| IBIS file stm32h562_563_573_lqfp100.ibs
[IBIS ver] 4.2
[File name] stm32h562_563_573_lqfp100.ibs
[File Rev] 1.1
[Date] 07-05-2024
[Source] Data Created at STMicroelectronics
[Notes]  File originated from ELDO simulations.
[Disclaimer]  This information is for modeling purpose only and is
   not guaranteed. The information is subject to change without
   notice.
[Copyright] Copyright 2024 STMicroelectronics Inc.
|   Component stm32h562_563_573_lqfp100
[Component] stm32h562_563_573_lqfp100
[Manufacturer] STMicroelectronics
[Package]
| variable   typ   min   max
R_pkg  0  NA  NA
L_pkg  0  NA  NA
C_pkg  0  NA  NA
[Pin]   signal_name   model_name
1  PE2  io8_ft_i3c_spi
2  PE3  io8_ft_i3c_spi
3  PE4  io8_ft_i3c_spi
4  PE5  io8_ft_i3c_spi
5  PE6  io8_ft_i3c_spi
6  VBAT  power
7  PC13  io8_ft_i3c_spi
8  PC14-OSC32_IN  io8_ft_i3c_spi
9  PC15-OSC32_OUT  io8_ft_i3c_spi
10  VSS  gnd
11  VDD  power
12  PH0-OSC_IN  io8_ft_i3c_spi
13  PH1-OSC_OUT  io8_ft_i3c_spi
14  NRST  ioreset_ft_v33
15  PC0  io8_ft_spi
16  PC1  io8_ft_spi
17  PC2  io8_ft_spi
18  PC3  io8_ft_spi
19  VSSA  nc
20  VREFM  nc
21  VREFP  nc
22  VDDA  nc
23  PA0  io8_ft_spi
24  PA1  io8_ft_spi_tamp
25  PA2  io8_ft_spi
26  PA3  io8_ft_spi
27  VSS  gnd
28  VDD  power
29  PA4  io8_ft_spi
30  PA5  io8_ft_spi
31  PA6  io8_ft_spi
32  PA7  io8_ft_spi
33  PC4  io8_ft_spi
34  PC5  io8_ft_spi
35  PB0  io8_ft_spi
36  PB1  io8_ft_spi
37  PB2  io8_ft_i3c_spi
38  PE7  io8_ft_i3c_spi
39  PE8  io8_ft_i3c_spi
40  PE9  io8_ft_i3c_spi
41  PE10  io8_ft_i3c_spi
42  PE11  io8_ft_i3c_spi
43  PE12  io8_ft_i3c_spi
44  PE13  io8_ft_i3c_spi
45  PE14  io8_ft_i3c_spi
46  PE15  io8_ft_i3c_spi
47  PB10  io8_ft_i3c_spi
48  VCAP  nc
49  VSS  gnd
50  VDD  power
51  PB12  io8_ft_i3c_spi
52  PB13  nc
|io8usb_ft_pd
53  PB14  nc
|io8usb_ft_pd
54  PB15  io8_ft_spi
55  PD8  io8_ft_i3c_spi
56  PD9  io8_ft_i3c_spi
57  PD10  io8_ft_i3c_spi
58  PD11  io8_ft_i3c_spi
59  PD12  io8_ft_i3c_spi
60  PD13  io8_ft_i3c_spi
61  PD14  io8_ft_i3c_spi
62  PD15  io8_ft_i3c_spi
63  PC6  io8_ft_i3c_spi
64  PC7  io8_ft_i3c_spi
65  PC8  io8_ft_i3c_spi
66  PC9  io8_ft_i3c_spi
67  PA8  io8_ft_i3c_spi
68  PA9  io8_ft_i3c_spi
69  PA10  io8_ft_i3c_spi
70  PA11  io8usb_ft_i3c_spi_phy
71  PA12  io8usb_ft_i3c_spi_phy
72  PA13  io8_ft_i3c_spi
73  VDD33_USB  power
74  VSS  gnd
75  VDD  power
76  PA14  io8_ft_i3c_spi
77  PA15  io8_ft_i3c_spi
78  PC10  io8_ft_i3c_spi
79  PC11  io8_ft_i3c_spi
80  PC12  io8_ft_i3c_spi
81  PD0  io8_ft_i3c_spi
82  PD1  io8_ft_i3c_spi
83  PD2  io8_ft_i3c_spi
84  PD3  io8_ft_i3c_spi
85  PD4  io8_ft_i3c_spi
86  PD5  io8_ft_i3c_spi
87  PD6  io8_ft_i3c_spi
88  PD7  io8_ft_i3c_spi
89  PB3  io8_ft_i3c_spi
90  PB4  io8_ft_i3c_spi
91  PB5  io8_ft_i3c_spi
92  PB6  io8_ft_i3c_spi
93  PB7  io8_ft_i3c_spi
94  BOOT0  vpphv
95  PB8  io8_ft_i3c_spi
96  PB9  io8_ft_i3c_spi
97  PE0  io8_ft_i3c_spi
98  VCAP  nc
99  VSS  gnd
100  VDD  power
[Package Model]   484-lqfp-14x14-100-ldo-221014
[Pin Mapping]   pulldown_ref   pullup_ref   | Comment
1  gndio  vddiom
2  gndio  vddiom
3  gndio  vddiom
4  gndio  vddiom
5  gndio  vddiom
6  nc  vsw
7  gndio  vddiom  | Depending on IO usage
| 7  gndio  vsw  | Depending on IO usage
8  gndio  vddiom  | Depending on IO usage
| 8  gndio  vsw  | Depending on IO usage
9  gndio  vddiom  | Depending on IO usage
| 9  gndio  vsw  | Depending on IO usage
10  gndio  nc
11  nc  vddiom
12  gndio  vddiom
13  gndio  vddiom
14  gndio  vddiom
15  gndio  vddiom
16  gndio  vddiom
17  gndio  vddiom
18  gndio  vddiom
19  nc  nc
20  nc  nc
21  nc  nc
22  nc  nc
23  gndio  vddiom
24  gndio  vddiom
25  gndio  vddiom
26  gndio  vddiom
27  gndio  nc
28  nc  vddiom
29  gndio  vddiom
30  gndio  vddiom
31  gndio  vddiom
32  gndio  vddiom
33  gndio  vddiom
34  gndio  vddiom
35  gndio  vddiom
36  gndio  vddiom
37  gndio  vddiom
38  gndio  vddiom
39  gndio  vddiom
40  gndio  vddiom
41  gndio  vddiom
42  gndio  vddiom
43  gndio  vddiom
44  gndio  vddiom
45  gndio  vddiom
46  gndio  vddiom
47  gndio  vddiom
48  nc  nc
49  gndio  nc
50  nc  vddiom
51  gndio  vddiom
|52  gndio  vddiom
|53  gndio  vddiom
52  nc  nc
53  nc  nc
54  gndio  vddiom
55  gndio  vddiom
56  gndio  vddiom
57  gndio  vddiom
58  gndio  vddiom
59  gndio  vddiom
60  gndio  vddiom
61  gndio  vddiom
62  gndio  vddiom
63  gndio  vddiom
64  gndio  vddiom
65  gndio  vddiom
66  gndio  vddiom
67  gndio  vddiom
68  gndio  vddiom  | Depending on IO usage
| 68  gndio  vddusb  | Depending on IO usage
69  gndio  vddiom  | Depending on IO usage
| 69  gndio  vddusb  | Depending on IO usage
70  gndio  vddiom  | Depending on IO usage
| 70  gndio  vddusb  | Depending on IO usage
71  gndio  vddiom  | Depending on IO usage
| 71  gndio  vddusb  | Depending on IO usage
72  gndio  vddiom  | Depending on IO usage
| 72  gndio  vddusb  | Depending on IO usage
73  nc  vddusb
74  gndio  nc
75  nc  vddiom
76  gndio  vddiom
77  gndio  vddiom
78  gndio  vddiom
79  gndio  vddiom
80  gndio  vddiom
81  gndio  vddiom
82  gndio  vddiom
83  gndio  vddiom
84  gndio  vddiom
85  gndio  vddiom
86  gndio  vddiom
87  gndio  vddiom
88  gndio  vddiom
89  gndio  vddiom
90  gndio  vddiom
91  gndio  vddiom
92  gndio  vddiom
93  gndio  vddiom
94  gndio  vddiom
95  gndio  vddiom
96  gndio  vddiom
97  gndio  vddiom
98  nc  nc
99  gndio  nc
100  nc  vddiom
[Model Selector] io8_ft_i3c_spi
io8_ft_spi_ls_1v2 "io8_ft spi low speed @ 1.2V"
io8_ft_spi_ls_1v8 "io8_ft spi low speed @ 1.8V"
io8_ft_spi_ls_3v3 "io8_ft spi low speed @ 3.3V"
io8_ft_spi_ms_1v2 "io8_ft spi med speed @ 1.2V"
io8_ft_spi_ms_1v8 "io8_ft spi med speed @ 1.8V"
io8_ft_spi_ms_3v3 "io8_ft spi med speed @ 3.3V"
io8_ft_spi_fs_1v2 "io8_ft spi fast speed @ 1.2V"
io8_ft_spi_fs_1v8 "io8_ft spi fast speed @ 1.8V"
io8_ft_spi_fs_3v3 "io8_ft spi fast speed @ 3.3V"
io8_ft_spi_hs_1v2 "io8_ft spi high speed @ 1.2V"
io8_ft_spi_hs_1v8 "io8_ft spi high speed @ 1.8V"
io8_ft_spi_hs_3v3 "io8_ft spi high speed @ 3.3V"
io8_ft_hslv_spi_ls_1v2 "io8_ft spi hslv low speed @ 1.2V"
io8_ft_hslv_spi_ls_1v8 "io8_ft spi hslv low speed @ 1.8V"
io8_ft_hslv_spi_ls_2v5 "io8_ft spi hslv low speed @ 2.5V"
io8_ft_hslv_spi_ms_1v2 "io8_ft spi hslv med speed @ 1.2V"
io8_ft_hslv_spi_ms_1v8 "io8_ft spi hslv med speed @ 1.8V"
io8_ft_hslv_spi_ms_2v5 "io8_ft spi hslv med speed @ 2.5V"
io8_ft_hslv_spi_fs_1v2 "io8_ft spi hslv fast speed @ 1.2V"
io8_ft_hslv_spi_fs_1v8 "io8_ft spi hslv fast speed @ 1.8V"
io8_ft_hslv_spi_fs_2v5 "io8_ft spi hslv fast speed @ 2.5V"
io8_ft_hslv_spi_hs_1v2 "io8_ft spi hslv high speed @ 1.2V"
io8_ft_hslv_spi_hs_1v8 "io8_ft spi hslv high speed @ 1.8V"
io8_ft_hslv_spi_hs_2v5 "io8_ft spi hslv high speed @ 2.5V"
io8_ft_i3c_spi_ls_1v2 "io8_ft i3c spi open-drain low speed @ 1.2V"
io8_ft_i3c_spi_ls_1v8 "io8_ft i3c spi open-drain low speed @ 1.8V"
io8_ft_i3c_spi_ls_3v3 "io8_ft i3c spi open-drain low speed @ 3.3V"
io8_ft_i3c_spi_ms_1v2 "io8_ft i3c spi open-drain med speed @ 1.2V"
io8_ft_i3c_spi_ms_1v8 "io8_ft i3c spi open-drain med speed @ 1.8V"
io8_ft_i3c_spi_ms_3v3 "io8_ft i3c spi open-drain med speed @ 3.3V"
io8_ft_i3c_spi_fs_1v2 "io8_ft i3c spi open-drain fast speed @ 1.2V"
io8_ft_i3c_spi_fs_1v8 "io8_ft i3c spi open-drain fast speed @ 1.8V"
io8_ft_i3c_spi_fs_3v3 "io8_ft i3c spi open-drain fast speed @ 3.3V"
io8_ft_i3c_spi_hs_1v2 "io8_ft i3c spi open-drain high speed @ 1.2V"
io8_ft_i3c_spi_hs_1v8 "io8_ft i3c spi open-drain high speed @ 1.8V"
io8_ft_i3c_spi_hs_3v3 "io8_ft i3c spi open-drain high speed @ 3.3V"
io8_ft_hslv_i3c_spi_ls_1v2 "io8_ft hslv i3c spi open-drain low speed @ 1.2V"
io8_ft_hslv_i3c_spi_ls_1v8 "io8_ft hslv i3c spi open-drain low speed @ 1.8V"
io8_ft_hslv_i3c_spi_ls_2v5 "io8_ft hslv i3c spi open-drain low speed @ 2.5V"
io8_ft_hslv_i3c_spi_ms_1v2 "io8_ft hslv i3c spi open-drain med speed @ 1.2V"
io8_ft_hslv_i3c_spi_ms_1v8 "io8_ft hslv i3c spi open-drain med speed @ 1.8V"
io8_ft_hslv_i3c_spi_ms_2v5 "io8_ft hslv i3c spi open-drain med speed @ 2.5V"
io8_ft_hslv_i3c_spi_fs_1v2 "io8_ft hslv i3c spi open-drain fast speed @ 1.2V"
io8_ft_hslv_i3c_spi_fs_1v8 "io8_ft hslv i3c spi open-drain fast speed @ 1.8V"
io8_ft_hslv_i3c_spi_fs_2v5 "io8_ft hslv i3c spi open-drain fast speed @ 2.5V"
io8_ft_hslv_i3c_spi_hs_1v2 "io8_ft hslv i3c spi open-drain high speed @ 1.2V"
io8_ft_hslv_i3c_spi_hs_1v8 "io8_ft hslv i3c spi open-drain high speed @ 1.8V"
io8_ft_hslv_i3c_spi_hs_2v5 "io8_ft hslv i3c spi open-drain high speed @ 2.5V"
io8_ft_i3c_fmp_spi_3v3 "io8_ft i3c fm+ spi open-drain @ 3.3V"
io8_ft_i3c_fmp_spi_1v8 "io8_ft i3c fm+ spi open-drain @ 1.8V"
io8_ft_i3c_fmp_spi_1v2 "io8_ft i3c fm+ spi open-drain @ 1.2V"
[Model Selector] io8_ft_spi
io8_ft_spi_ls_1v2 "io8_ft spi low speed @ 1.2V"
io8_ft_spi_ls_1v8 "io8_ft spi low speed @ 1.8V"
io8_ft_spi_ls_3v3 "io8_ft spi low speed @ 3.3V"
io8_ft_spi_ms_1v2 "io8_ft spi med speed @ 1.2V"
io8_ft_spi_ms_1v8 "io8_ft spi med speed @ 1.8V"
io8_ft_spi_ms_3v3 "io8_ft spi med speed @ 3.3V"
io8_ft_spi_fs_1v2 "io8_ft spi fast speed @ 1.2V"
io8_ft_spi_fs_1v8 "io8_ft spi fast speed @ 1.8V"
io8_ft_spi_fs_3v3 "io8_ft spi fast speed @ 3.3V"
io8_ft_spi_hs_1v2 "io8_ft spi high speed @ 1.2V"
io8_ft_spi_hs_1v8 "io8_ft spi high speed @ 1.8V"
io8_ft_spi_hs_3v3 "io8_ft spi high speed @ 3.3V"
io8_ft_hslv_spi_ls_1v2 "io8_ft spi hslv low speed @ 1.2V"
io8_ft_hslv_spi_ls_1v8 "io8_ft spi hslv low speed @ 1.8V"
io8_ft_hslv_spi_ls_2v5 "io8_ft spi hslv low speed @ 2.5V"
io8_ft_hslv_spi_ms_1v2 "io8_ft spi hslv med speed @ 1.2V"
io8_ft_hslv_spi_ms_1v8 "io8_ft spi hslv med speed @ 1.8V"
io8_ft_hslv_spi_ms_2v5 "io8_ft spi hslv med speed @ 2.5V"
io8_ft_hslv_spi_fs_1v2 "io8_ft spi hslv fast speed @ 1.2V"
io8_ft_hslv_spi_fs_1v8 "io8_ft spi hslv fast speed @ 1.8V"
io8_ft_hslv_spi_fs_2v5 "io8_ft spi hslv fast speed @ 2.5V"
io8_ft_hslv_spi_hs_1v2 "io8_ft spi hslv high speed @ 1.2V"
io8_ft_hslv_spi_hs_1v8 "io8_ft spi hslv high speed @ 1.8V"
io8_ft_hslv_spi_hs_2v5 "io8_ft spi hslv high speed @ 2.5V"
[Model Selector] io8_ft_spi_tamp
io8_ft_spi_ls_1v2 "io8_ft spi low speed @ 1.2V"
io8_ft_spi_ls_1v8 "io8_ft spi low speed @ 1.8V"
io8_ft_spi_ls_3v3 "io8_ft spi low speed @ 3.3V"
io8_ft_spi_ms_1v2 "io8_ft spi med speed @ 1.2V"
io8_ft_spi_ms_1v8 "io8_ft spi med speed @ 1.8V"
io8_ft_spi_ms_3v3 "io8_ft spi med speed @ 3.3V"
io8_ft_spi_fs_1v2 "io8_ft spi fast speed @ 1.2V"
io8_ft_spi_fs_1v8 "io8_ft spi fast speed @ 1.8V"
io8_ft_spi_fs_3v3 "io8_ft spi fast speed @ 3.3V"
io8_ft_spi_hs_1v2 "io8_ft spi high speed @ 1.2V"
io8_ft_spi_hs_1v8 "io8_ft spi high speed @ 1.8V"
io8_ft_spi_hs_3v3 "io8_ft spi high speed @ 3.3V"
io8_ft_hslv_spi_ls_1v2 "io8_ft spi hslv low speed @ 1.2V"
io8_ft_hslv_spi_ls_1v8 "io8_ft spi hslv low speed @ 1.8V"
io8_ft_hslv_spi_ls_2v5 "io8_ft spi hslv low speed @ 2.5V"
io8_ft_hslv_spi_ms_1v2 "io8_ft spi hslv med speed @ 1.2V"
io8_ft_hslv_spi_ms_1v8 "io8_ft spi hslv med speed @ 1.8V"
io8_ft_hslv_spi_ms_2v5 "io8_ft spi hslv med speed @ 2.5V"
io8_ft_hslv_spi_fs_1v2 "io8_ft spi hslv fast speed @ 1.2V"
io8_ft_hslv_spi_fs_1v8 "io8_ft spi hslv fast speed @ 1.8V"
io8_ft_hslv_spi_fs_2v5 "io8_ft spi hslv fast speed @ 2.5V"
io8_ft_hslv_spi_hs_1v2 "io8_ft spi hslv high speed @ 1.2V"
io8_ft_hslv_spi_hs_1v8 "io8_ft spi hslv high speed @ 1.8V"
io8_ft_hslv_spi_hs_2v5 "io8_ft spi hslv high speed @ 2.5V"
io8_ft_tamp_v33_1v2 "io8_ft tamp V33 @ 1.2V"
io8_ft_tamp_v33_1v8 "io8_ft tamp V33 @ 1.2V"
io8_ft_tamp_v33_3v3 "io8_ft tamp V33 @ 1.2V"
[Model Selector] io8usb_ft_i3c_spi_phy
io8_ft_spi_ls_1v2 "io8_ft spi low speed @ 1.2V"
io8_ft_spi_ls_1v8 "io8_ft spi low speed @ 1.8V"
io8_ft_spi_ls_3v3 "io8_ft spi low speed @ 3.3V"
io8_ft_spi_ms_1v2 "io8_ft spi med speed @ 1.2V"
io8_ft_spi_ms_1v8 "io8_ft spi med speed @ 1.8V"
io8_ft_spi_ms_3v3 "io8_ft spi med speed @ 3.3V"
io8_ft_spi_fs_1v2 "io8_ft spi fast speed @ 1.2V"
io8_ft_spi_fs_1v8 "io8_ft spi fast speed @ 1.8V"
io8_ft_spi_fs_3v3 "io8_ft spi fast speed @ 3.3V"
io8_ft_spi_hs_1v2 "io8_ft spi high speed @ 1.2V"
io8_ft_spi_hs_1v8 "io8_ft spi high speed @ 1.8V"
io8_ft_spi_hs_3v3 "io8_ft spi high speed @ 3.3V"
io8_ft_hslv_spi_ls_1v2 "io8_ft spi hslv low speed @ 1.2V"
io8_ft_hslv_spi_ls_1v8 "io8_ft spi hslv low speed @ 1.8V"
io8_ft_hslv_spi_ls_2v5 "io8_ft spi hslv low speed @ 2.5V"
io8_ft_hslv_spi_ms_1v2 "io8_ft spi hslv med speed @ 1.2V"
io8_ft_hslv_spi_ms_1v8 "io8_ft spi hslv med speed @ 1.8V"
io8_ft_hslv_spi_ms_2v5 "io8_ft spi hslv med speed @ 2.5V"
io8_ft_hslv_spi_fs_1v2 "io8_ft spi hslv fast speed @ 1.2V"
io8_ft_hslv_spi_fs_1v8 "io8_ft spi hslv fast speed @ 1.8V"
io8_ft_hslv_spi_fs_2v5 "io8_ft spi hslv fast speed @ 2.5V"
io8_ft_hslv_spi_hs_1v2 "io8_ft spi hslv high speed @ 1.2V"
io8_ft_hslv_spi_hs_1v8 "io8_ft spi hslv high speed @ 1.8V"
io8_ft_hslv_spi_hs_2v5 "io8_ft spi hslv high speed @ 2.5V"
io8_ft_i3c_spi_ls_1v2 "io8_ft i3c spi open-drain low speed @ 1.2V"
io8_ft_i3c_spi_ls_1v8 "io8_ft i3c spi open-drain low speed @ 1.8V"
io8_ft_i3c_spi_ls_3v3 "io8_ft i3c spi open-drain low speed @ 3.3V"
io8_ft_i3c_spi_ms_1v2 "io8_ft i3c spi open-drain med speed @ 1.2V"
io8_ft_i3c_spi_ms_1v8 "io8_ft i3c spi open-drain med speed @ 1.8V"
io8_ft_i3c_spi_ms_3v3 "io8_ft i3c spi open-drain med speed @ 3.3V"
io8_ft_i3c_spi_fs_1v2 "io8_ft i3c spi open-drain fast speed @ 1.2V"
io8_ft_i3c_spi_fs_1v8 "io8_ft i3c spi open-drain fast speed @ 1.8V"
io8_ft_i3c_spi_fs_3v3 "io8_ft i3c spi open-drain fast speed @ 3.3V"
io8_ft_i3c_spi_hs_1v2 "io8_ft i3c spi open-drain high speed @ 1.2V"
io8_ft_i3c_spi_hs_1v8 "io8_ft i3c spi open-drain high speed @ 1.8V"
io8_ft_i3c_spi_hs_3v3 "io8_ft i3c spi open-drain high speed @ 3.3V"
io8_ft_hslv_i3c_spi_ls_1v2 "io8_ft hslv i3c spi open-drain low speed @ 1.2V"
io8_ft_hslv_i3c_spi_ls_1v8 "io8_ft hslv i3c spi open-drain low speed @ 1.8V"
io8_ft_hslv_i3c_spi_ls_2v5 "io8_ft hslv i3c spi open-drain low speed @ 2.5V"
io8_ft_hslv_i3c_spi_ms_1v2 "io8_ft hslv i3c spi open-drain med speed @ 1.2V"
io8_ft_hslv_i3c_spi_ms_1v8 "io8_ft hslv i3c spi open-drain med speed @ 1.8V"
io8_ft_hslv_i3c_spi_ms_2v5 "io8_ft hslv i3c spi open-drain med speed @ 2.5V"
io8_ft_hslv_i3c_spi_fs_1v2 "io8_ft hslv i3c spi open-drain fast speed @ 1.2V"
io8_ft_hslv_i3c_spi_fs_1v8 "io8_ft hslv i3c spi open-drain fast speed @ 1.8V"
io8_ft_hslv_i3c_spi_fs_2v5 "io8_ft hslv i3c spi open-drain fast speed @ 2.5V"
io8_ft_hslv_i3c_spi_hs_1v2 "io8_ft hslv i3c spi open-drain high speed @ 1.2V"
io8_ft_hslv_i3c_spi_hs_1v8 "io8_ft hslv i3c spi open-drain high speed @ 1.8V"
io8_ft_hslv_i3c_spi_hs_2v5 "io8_ft hslv i3c spi open-drain high speed @ 2.5V"
io8_ft_i3c_fmp_spi_3v3 "io8_ft i3c fm+ spi open-drain @ 3.3V"
io8_ft_i3c_fmp_spi_1v8 "io8_ft i3c fm+ spi open-drain @ 1.8V"
io8_ft_i3c_fmp_spi_1v2 "io8_ft i3c fm+ spi open-drain @ 1.2V"
io8usb_ft_phy_ls_2v5 "iousb ft low speed @ 2.5V"
io8usb_ft_phy_ls_3v3 "iousb ft low speed @ 3.3V"
io8usb_ft_phy_fs_2v5 "iousb ft fast speed @ 2.5V"
io8usb_ft_phy_fs_3v3 "iousb ft fast speed @ 3.3V"
[Model Selector] ioreset_ft_v33
ioreset_ft_v33_1v2 "Reset PAD. 5V tolerant. 1.2V range"
ioreset_ft_v33_1v8 "Reset PAD. 5V tolerant. 1.8V range"
ioreset_ft_v33_3v3 "Reset PAD. 5V tolerant. 3.3V range"
[Model Selector] vpphv
vpphv_1v2 "Flash Test cell v33 = 1.2 V range"
vpphv_1v8 "Flash Test cell v33 = 1.8 V range"
vpphv_3v3 "Flash Test cell v33 = 3.3 V range"
[Define Package Model]  484-lqfp-14x14-100-ldo-221014
[Manufacturer]  Unknown
[OEM]  Unknown
[Description]  None
[Number Of Pins]  96
[Pin Numbers]
| Pin Num   Terminal Name
14 | NRST
23 | PA0
24 | PA1
25 | PA2
26 | PA3
29 | PA4
30 | PA5
31 | PA6
32 | PA7
67 | PA8
68 | PA9
69 | PA10
70 | PA11
71 | PA12
72 | PA13
76 | PA14
77 | PA15
35 | PB0
36 | PB1
37 | PB2
89 | PB3
90 | PB4
91 | PB5
92 | PB6
93 | PB7
95 | PB8
96 | PB9
47 | PB10
51 | PB12
52 | PB13
53 | PB14
54 | PB15
15 | PC0
16 | PC1
17 | PC2
18 | PC3
33 | PC4
34 | PC5
63 | PC6
64 | PC7
65 | PC8
66 | PC9
78 | PC10
79 | PC11
80 | PC12
7 | PC13
8 | PC14-OSC32_IN
9 | PC15-OSC32_OUT
81 | PD0
82 | PD1
83 | PD2
84 | PD3
85 | PD4
86 | PD5
87 | PD6
88 | PD7
55 | PD8
56 | PD9
57 | PD10
58 | PD11
59 | PD12
60 | PD13
61 | PD14
62 | PD15
97 | PE0
1 | PE2
2 | PE3
3 | PE4
4 | PE5
5 | PE6
38 | PE7
39 | PE8
40 | PE9
41 | PE10
42 | PE11
43 | PE12
44 | PE13
45 | PE14
46 | PE15
12 | PH0-OSC_IN
13 | PH1-OSC_OUT
6 | VBAT
48 | VCAP
98 | VCAP
50 | VDD
75 | VDD
11 | VDD
28 | VDD
100 | VDD
73 | VDD33_USB
22 | VDDA
94 | BOOT0
20 | VREFM
21 | VREFP
10 | VSS
19 | VSSA
|[Merged Pins]  10
|27  |  VSS
|49  |  VSS
|74  |  VSS
|99  |  VSS
[Model Data]
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[End Model Data]
[End Package Model]
|End [Component]
| Models and submodels in the file (64): io8_ft_hslv_i3c_spi_fs_1v2 (I/O_open_drain), io8_ft_hslv_i3c_spi_fs_1v8 (I/O_open_drain), io8_ft_hslv_i3c_spi_fs_2v5 (I/O_open_drain), io8_ft_hslv_i3c_spi_hs_1v2 (I/O_open_drain), io8_ft_hslv_i3c_spi_hs_1v8 (I/O_open_drain), io8_ft_hslv_i3c_spi_hs_2v5 (I/O_open_drain), io8_ft_hslv_i3c_spi_ls_1v2 (I/O_open_drain), io8_ft_hslv_i3c_spi_ls_1v8 (I/O_open_drain), io8_ft_hslv_i3c_spi_ls_2v5 (I/O_open_drain), io8_ft_hslv_i3c_spi_ms_1v2 (I/O_open_drain), io8_ft_hslv_i3c_spi_ms_1v8 (I/O_open_drain), io8_ft_hslv_i3c_spi_ms_2v5 (I/O_open_drain), io8_ft_hslv_spi_fs_1v2 (I/O), io8_ft_hslv_spi_fs_1v8 (I/O), io8_ft_hslv_spi_fs_2v5 (I/O), io8_ft_hslv_spi_hs_1v2 (I/O), io8_ft_hslv_spi_hs_1v8 (I/O), io8_ft_hslv_spi_hs_2v5 (I/O), io8_ft_hslv_spi_ls_1v2 (I/O), io8_ft_hslv_spi_ls_1v8 (I/O), io8_ft_hslv_spi_ls_2v5 (I/O), io8_ft_hslv_spi_ms_1v2 (I/O), io8_ft_hslv_spi_ms_1v8 (I/O), io8_ft_hslv_spi_ms_2v5 (I/O), io8_ft_i3c_fmp_spi_1v2 (I/O_open_drain), io8_ft_i3c_fmp_spi_1v8 (I/O_open_drain), io8_ft_i3c_fmp_spi_3v3 (I/O_open_drain), io8_ft_i3c_spi_fs_1v2 (I/O_open_drain), io8_ft_i3c_spi_fs_1v8 (I/O_open_drain), io8_ft_i3c_spi_fs_3v3 (I/O_open_drain), io8_ft_i3c_spi_hs_1v2 (I/O_open_drain), io8_ft_i3c_spi_hs_1v8 (I/O_open_drain), io8_ft_i3c_spi_hs_3v3 (I/O_open_drain), io8_ft_i3c_spi_ls_1v2 (I/O_open_drain), io8_ft_i3c_spi_ls_1v8 (I/O_open_drain), io8_ft_i3c_spi_ls_3v3 (I/O_open_drain), io8_ft_i3c_spi_ms_1v2 (I/O_open_drain), io8_ft_i3c_spi_ms_1v8 (I/O_open_drain), io8_ft_i3c_spi_ms_3v3 (I/O_open_drain), io8_ft_spi_fs_1v2 (I/O), io8_ft_spi_fs_1v8 (I/O), io8_ft_spi_fs_3v3 (I/O), io8_ft_spi_hs_1v2 (I/O), io8_ft_spi_hs_1v8 (I/O), io8_ft_spi_hs_3v3 (I/O), io8_ft_spi_ls_1v2 (I/O), io8_ft_spi_ls_1v8 (I/O), io8_ft_spi_ls_3v3 (I/O), io8_ft_spi_ms_1v2 (I/O), io8_ft_spi_ms_1v8 (I/O), io8_ft_spi_ms_3v3 (I/O), io8_ft_tamp_v33_1v2 (I/O), io8_ft_tamp_v33_1v8 (I/O), io8_ft_tamp_v33_3v3 (I/O), io8usb_ft_phy_fs_2v5 (I/O), io8usb_ft_phy_fs_3v3 (I/O), io8usb_ft_phy_ls_2v5 (I/O), io8usb_ft_phy_ls_3v3 (I/O), ioreset_ft_v33_1v2 (I/O_open_drain), ioreset_ft_v33_1v8 (I/O_open_drain), ioreset_ft_v33_3v3 (I/O_open_drain), vpphv_1v2 (Input), vpphv_1v8 (Input), vpphv_3v3 (Input)
